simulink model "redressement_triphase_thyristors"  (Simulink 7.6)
settings: Solver=ode23tb  StartTime=0.0  StopTime=0.05  RelTol=1e-3
InitFcn:
  | clc
StopFcn:
  | close all, clc, clear all
  | load redressement_triphase.mat
  | plot(x(1,:),x(2,:))
  | hold on
  | plot(x(1,:),x(3,:))
  | plot(x(1,:),x(4,:))
  | %axis([0 0.14 -0.2 1.7])
  | grid
  | title('Signaux aux cathodes, anodes et signal redressé')
  | xlabel('temps')
  | 
  | load phases.mat
  | figure
  | plot(y(1,:),y(2,:),'o')
  | hold on
  | plot(y(1,:),y(3,:),'+')
  | plot(y(1,:),y(4,:),'*')
  | axis([0 0.002 -400 400])
  | grid
libraries: powerlib x20, powerlib_extras x1

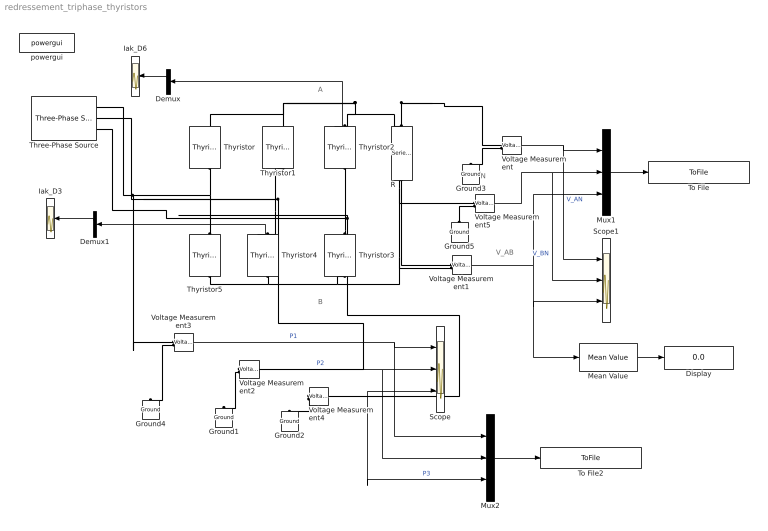
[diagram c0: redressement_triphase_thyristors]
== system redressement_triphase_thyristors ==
  note: A
  note: B
  note: N
  note: V_AB
  Demux : Demux  Outputs=2
  Demux1 : Demux  Outputs=2
  Display : Display
  Ground{1..5} (5 alike) : powerlib/Elements/Ground  DialogController=POWERSYS.PowerSysDialog  PhysicalDomain=powersysdomain  SubClassName=unknown  LeftPortType=p1  RightPortType=p1  LConnTagsString=a
  Iak_D3 : Scope
  Iak_D6 : Scope
  Mean Value : powerlib_extras/Measurements/Mean Value  DialogController=POWERSYS.PowerSysDialog  SystemSampleTime=-1  Period=1/60
  Mux1 : Mux  Inputs=3
  Mux2 : Mux  Inputs=3
  R : powerlib/Elements/Series RLC Branch  DialogController=POWERSYS.PowerSysDialog  PhysicalDomain=powersysdomain  SubClassName=unknown  LeftPortType=p1  RightPortType=p1  LConnTagsString=__new0  RConnTagsString=__new0  BranchType=R  Resistance=12e3  Inductance=1e-3  SetiL0=off  InitialCurrent=0  Capacitance=1e-6  Setx0=off  InitialVoltage=0  Measurements=None
  Scope : Scope  NumInputPorts=3
  Scope1 : Scope  NumInputPorts=3
  Three-Phase Source : powerlib/Electrical Sources/Three-Phase Source  DialogController=POWERSYS.PowerSysDialog  SystemSampleTime=-1  Voltage=380  PhaseAngle=0  Frequency=60  InternalConnection=Yg  SpecifyImpedance=off  Resistance=0.8929  Inductance=16.58e-3  ShortCircuitLevel=100e6  BaseVoltage=25e3  XRratio=7
  Thyristor{,1..5} (6 alike) : powerlib/Power Electronics/Thyristor  DialogController=POWERSYS.PowerSysDialog  SystemSampleTime=-1  Ron=0.001  Lon=0  Vf=0.8  IC=0  Rs=500  Cs=250e-9  Measurements=on
  To File : ToFile  Filename=redressement_triphase  MatrixName=x
  To File2 : ToFile  Filename=phases  MatrixName=y
  Voltage Measurement{,1..5} (6 alike) : powerlib/Measurements/Voltage Measurement  DialogController=POWERSYS.PowerSysDialog  SystemSampleTime=-1  PhasorSimulation=off  OutputType=Complex  PSBequivalent=0
  powergui : powerlib/powergui  SystemSampleTime=-1  SimulationMode=Continuous  SampleTime=0  frequency=60  SPID=off  DisableSnubberDevices=off  DisableRonSwitches=off  DisableVfSwitches=off  SwTol=0  Interpol=off  frequencyindice=0  echomessages=off  HookPort=off  DisplayEquations=off  FunctionMessages=off  EnableUseOfTLC=off  x0status=blocks  RestoreLinks=warning  ResistiveCurrentMeasurement=off  Frange=[0:2:500]  Ylog=off  Xlog=on  ShowGrid=off  save=off  variable=ZData  ZoomFFT=on  StartTime=0.0  cycles=1  DisplayStyle=1  fundamental=60  FreqAxis=off  MaxFrequency=1000  frequencyindicesteady=60  RmsSteady=1  display=off  Ts=0  methode=off
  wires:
  Voltage Measurement4/1 -> Scope/3, Mux2/3  "P3"
  Voltage Measurement2/1 -> Scope/2, Mux2/2  "P2"
  Voltage Measurement3/1 -> Scope/1, Mux2/1  "P1"
  Voltage Measurement/1 -> Mux1/1, Scope1/1  "V_AN"
  Voltage Measurement5/1 -> Mux1/2, Scope1/2  "V_BN"
  Voltage Measurement1/1 -> Mux1/3, Scope1/3, Mean Value/1
  Mux1/1 -> To File/1
  Mux2/1 -> To File2/1
  Thyristor2/1 -> Demux/1
  Thyristor4/1 -> Demux1/1
  Demux/1 -> Iak_D6/1
  Demux1/1 -> Iak_D3/1
  Mean Value/1 -> Display/1
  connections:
  Thyristor5/RConn1 -- Three-Phase Source/RConn1 -- Voltage Measurement3/LConn1 -- Thyristor/LConn1
  Thyristor4/RConn1 -- Three-Phase Source/RConn2 -- Voltage Measurement2/LConn1 -- Thyristor1/LConn1
  Thyristor3/RConn1 -- Three-Phase Source/RConn3 -- Voltage Measurement4/LConn1 -- Thyristor2/LConn1
  Thyristor2/RConn1 -- Voltage Measurement/LConn1 -- Voltage Measurement1/LConn1 -- R/RConn1 -- Thyristor/RConn1 -- Thyristor1/RConn1
  Voltage Measurement2/LConn2 -- Ground1/LConn1
  Voltage Measurement3/LConn2 -- Ground4/LConn1
  Voltage Measurement4/LConn2 -- Ground2/LConn1
  Voltage Measurement/LConn2 -- Ground3/LConn1
  Ground5/LConn1 -- Voltage Measurement5/LConn2
  Thyristor5/LConn1 -- R/LConn1 -- Voltage Measurement5/LConn1 -- Voltage Measurement1/LConn2 -- Thyristor3/LConn1 -- Thyristor4/LConn1
